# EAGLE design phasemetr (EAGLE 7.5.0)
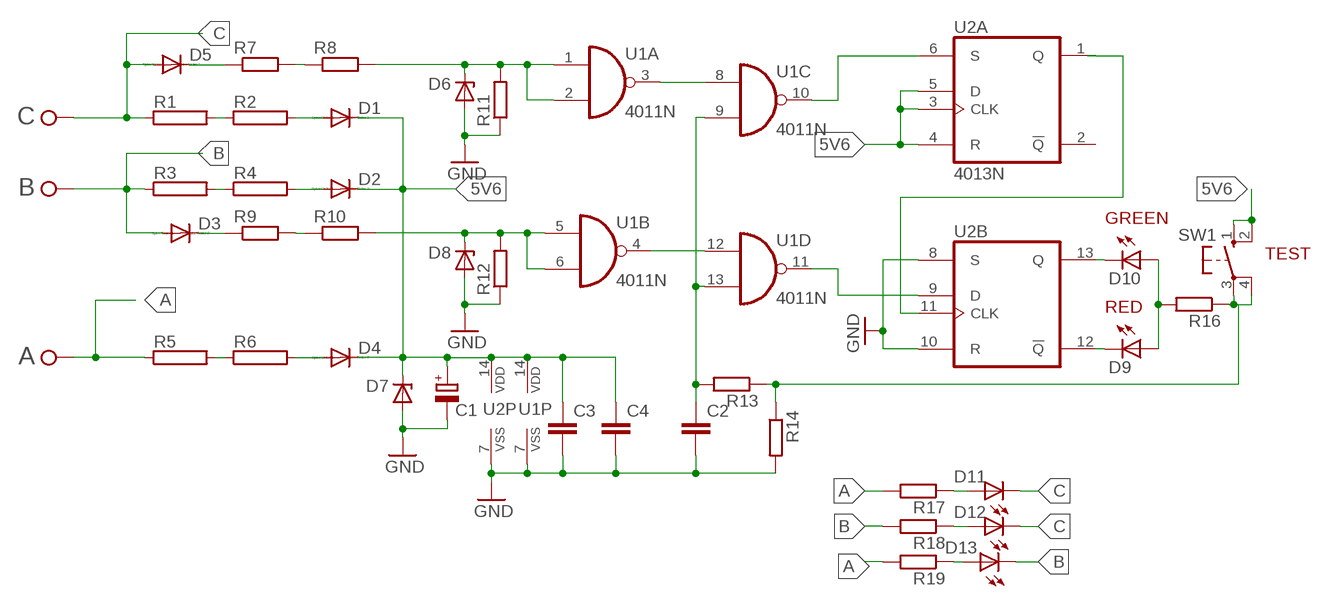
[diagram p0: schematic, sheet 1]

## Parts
A  TPPAD1-20  [P1-20]
B  TPPAD1-20  [P1-20]
C  TPPAD1-20  [P1-20]
C1  CPOL-EUE5-10.5  [E5-10,5]
C2  C-EUC1206  [C1206]
C3  C-EUC1206  [C1206]
C4  C-EUC1206  [C1206]
D1  1N4004  [DO41-10]
D2  1N4004  [DO41-10]
D3  1N4004  [DO41-10]
D4  1N4004  [DO41-10]
D5  1N4004  [DO41-10]
D6  ZY  [P1Z12]
D7  ZY  [P1Z12]
D8  ZY  [P1Z12]
D9  LED5MM  [LED5MM]
D10  LED5MM  [LED5MM]
D11  LED5MM  [LED5MM]
D12  LED5MM  [LED5MM]
D13  LED5MM  [LED5MM]
R1  RRWM8X34  [RWM8X34]
R2  RRWM8X34  [RWM8X34]
R3  RRWM8X34  [RWM8X34]
R4  RRWM8X34  [RWM8X34]
R5  RRWM8X34  [RWM8X34]
R6  RRWM8X34  [RWM8X34]
R7  R-EU_0309/12  [0309/12]
R8  R-EU_0309/12  [0309/12]
R9  R-EU_0309/12  [0309/12]
R10  R-EU_0309/12  [0309/12]
R11  R-EU_0309/12  [0309/12]
R12  R-EU_0309/12  [0309/12]
R13  R-EU_0309/12  [0309/12]
R14  R-EU_0309/12  [0309/12]
R16  R-EU_0309/12  [0309/12]
R17  R-EU_0309/12  [0309/12]
R18  R-EU_0309/12  [0309/12]
R19  R-EU_0309/12  [0309/12]
SW1  10-XX  [B3F-10XX]
U1  4011N  [DIL14]
U2  4013N  [DIL14]

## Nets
5V6: C1.+ C3.1 C4.1 D1.C D2.C D4.C D7.C SW1.1(S) SW1.2(S1) U1.14(P:VDD) U2.3(A:CLK) U2.4(A:R) U2.5(A:D) U2.14(P:VDD)
A: A.TP R5.1 R17.2 R19.2
B: B.TP D3.A D13.K(C) R3.1 R18.2
C: C.TP D5.A D11.K(C) D12.K(C) R1.1
GND: C1.- C2.2 C3.2 C4.2 D6.A D7.A D8.A R11.1 R12.1 R14.2 U1.7(P:VSS) U2.7(P:VSS) U2.8(B:S) U2.10(B:R)
N$2: D5.C R7.1
N$3: D11.A R17.1
N$4: R1.2 R2.1
N$5: D1.A R2.2
N$6: D2.A R4.2
N$7: R3.2 R4.1
N$9: R5.2 R6.1
N$10: D4.A R6.2
N$11: R7.2 R8.1
N$12: D3.C R9.1
N$13: R9.2 R10.1
N$14: D9.A D10.A R16.2
N$15: D6.C R8.2 R11.2 U1.1(A:I0) U1.2(A:I1)
N$16: U1.3(A:O) U1.8(C:I0)
N$17: U1.10(C:O) U2.6(A:S)
N$18: D8.C R10.2 R12.2 U1.5(B:I0) U1.6(B:I1)
N$20: U1.4(B:O) U1.12(D:I0)
N$21: C2.1 R13.2 U1.9(C:I1) U1.13(D:I1)
N$22: U1.11(D:O) U2.9(B:D)
N$23: U2.11(B:CLK)
N$24: D10.K(C) U2.13(B:Q)
N$25: D9.K(C) U2.12(B:!Q)
N$26: R13.1 R14.1 R16.1 SW1.3(P) SW1.4(P1)
N$27: D12.A R18.1
N$29: D13.A R19.1
Unconnected: U2.1(A:Q) U2.2(A:!Q)

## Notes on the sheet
- GREEN
- TEST
- RED

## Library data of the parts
A B C = testpad:TP: Test pad
C1 = rcl:CPOL-EU: POLARIZED CAPACITOR, European symbol
C2-C4 = rcl:C-EU: CAPACITOR, European symbol
D1-D5 = diode:1N4004: DIODE
D6-D8 = diode:ZY: Z DIODE
D9-D13 = led:LED: LED
R1-R6 = resistor-power:R: Power Resitor; OC_FARNELL: unknown; OC_NEWARK: unknown
R7-R14 R16-R19 = rcl:R-EU_: RESISTOR, European symbol
SW1 = switch-omron:10-XX: OMRON SWITCH; MPN: B3F-1000; OC_FARNELL: 176432; OC_NEWARK: 36M3542
U1 = 40xx:4011: Quad 2-input NAND
U2 = 40xx:4013: Dual D FLIP FLOP, set/reset

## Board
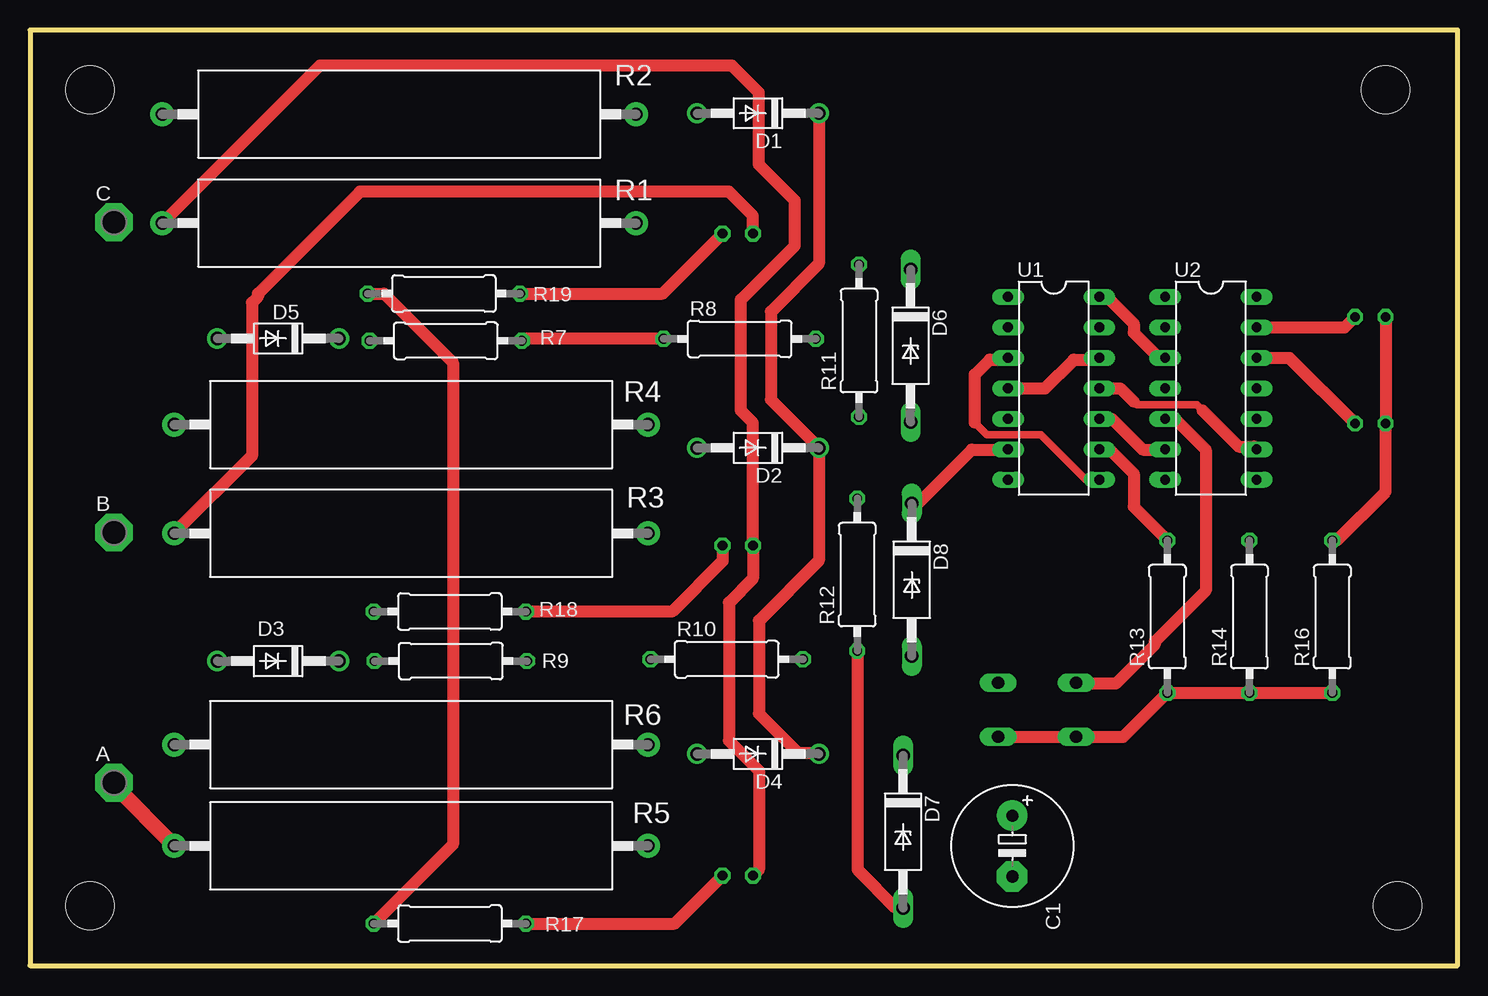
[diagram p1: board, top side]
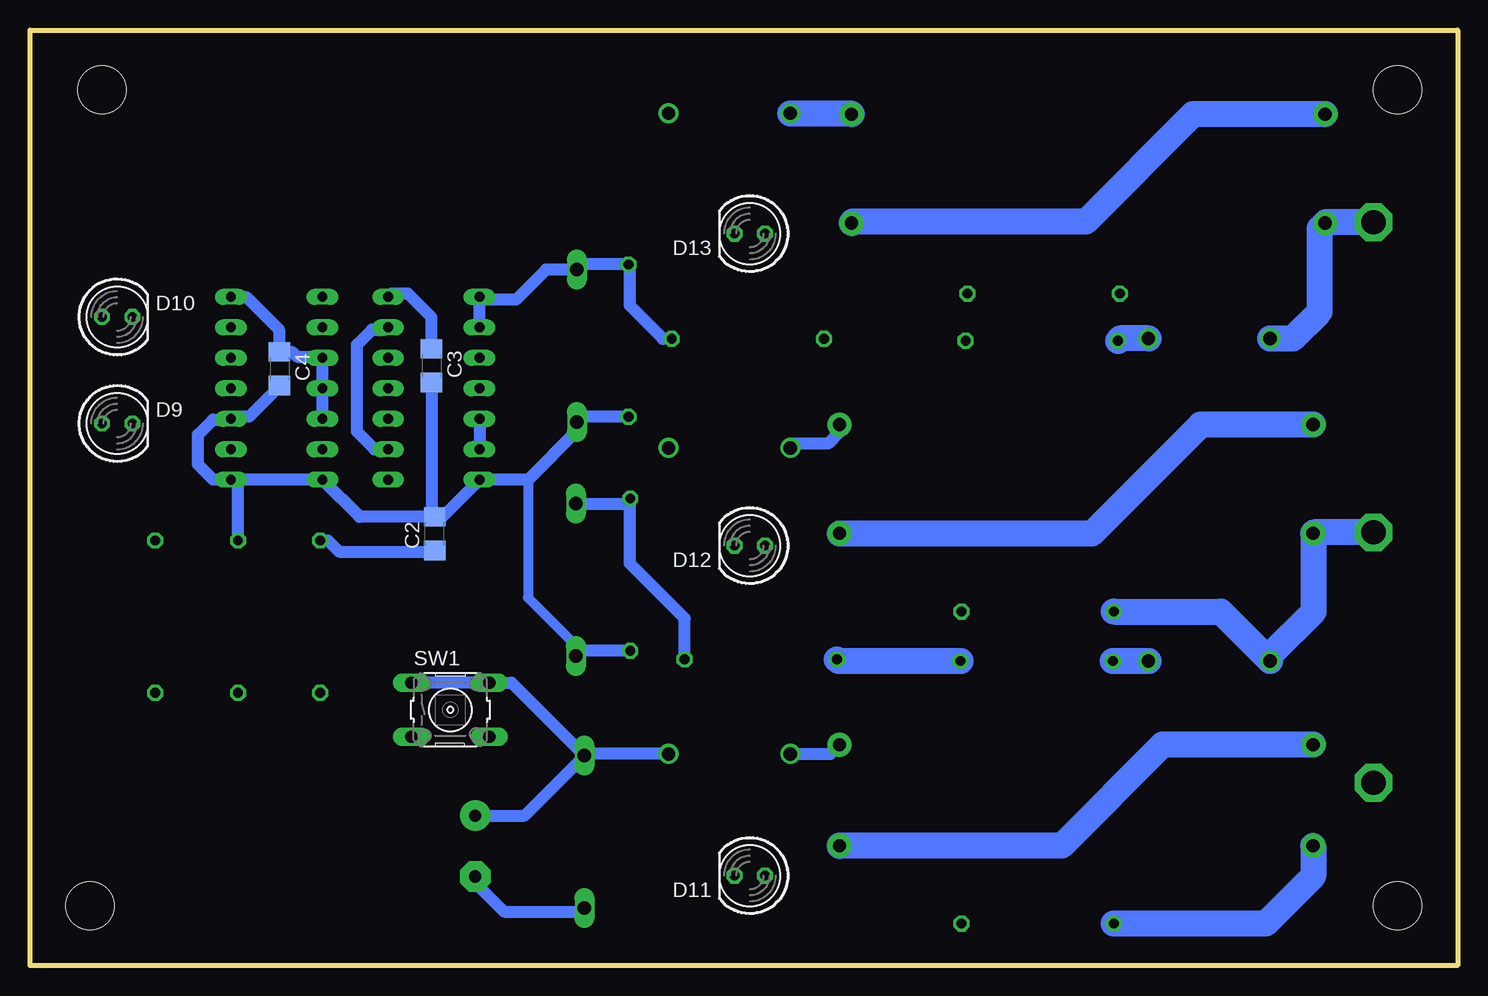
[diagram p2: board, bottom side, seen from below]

Size 119 x 77.97 mm. Coordinates in mm from the lower left corner, seen from the top.
Outline: 0,0 119,0 119,77.97 0,77.97 0,0
Copper layers (1*16): Top 0.035mm / dielectric 1.5mm / Bottom 0.035mm
Design rules "default": minimum track width 10mil, minimum drill 24mil, track to track 8mil, track to pad 8mil, pad to pad 8mil, via to via 8mil, smd to smd 8mil, copper to edge 40mil, drill to drill 8mil, minimum pad ring 10mil, minimum via ring 8mil, stop-mask expansion 4mil, vias tented up to drill 0mil, thermal gap 10mil
Holes 4 mm at 5,73 5,5 114,5 113,73

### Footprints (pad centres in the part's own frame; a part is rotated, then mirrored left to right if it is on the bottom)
P1-20 = drill 2.007 pad 3.15 octagon: TP 0,0
E5-10,5 = drill 1.016 pad 2.54: + -2.54,0 | drill 1.016 pad 2.54 octagon: - 2.54,0
C1206 = smd 1.6 x 1.8: 1 -1.4,0; 2 1.4,0
DO41-10 = drill 1.118: A 5.08,0; C -5.08,0
P1Z12 = drill 1.118 long: A 6.35,0; C -6.35,0
LED5MM = drill 0.813 octagon: A -1.27,0; K 1.27,0
RWM8X34 = drill 1.1 pad 2: 1 -19.74,0; 2 19.74,0
0309/12 = drill 0.813 octagon: 1 -6.35,0; 2 6.35,0
B3F-10XX = drill 1.016 long: 1 -3.251,2.261; 2 3.251,2.261; 3 -3.251,-2.261; 4 3.251,-2.261
DIL14 = drill 0.813 long: 1 -7.62,-3.81; 2 -5.08,-3.81; 3 -2.54,-3.81; 4 0,-3.81; 5 2.54,-3.81; 6 5.08,-3.81; 7 7.62,-3.81; 8 7.62,3.81; 9 5.08,3.81; 10 2.54,3.81; 11 0,3.81; 12 -2.54,3.81; 13 -5.08,3.81; 14 -7.62,3.81

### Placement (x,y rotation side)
A  7,15.25 0 top
B  7,36.1 0 top
C  7,61.95 0 top
C1  81.89,9.96 270 top
C2  85.26,36 90 bottom
C3  85.53,50 270 bottom
C4  98.2,49.75 270 bottom
D1  60.69,71.03 180 top
D2  60.69,43.15 180 top
D3  20.69,25.38 180 top
D4  60.69,17.64 180 top
D5  20.69,52.26 180 top
D6  73.4,51.65 270 top
D7  72.78,11.15 270 top
D8  73.5,32.15 270 top
D9  111.73,45.18 0 bottom
D10  111.73,54.06 0 bottom
D11  59,7.5 180 bottom
D12  59,35 180 bottom
D13  59,61 180 bottom
R1  30.78,61.88 0 top
R2  30.78,70.95 0 top
R3  31.78,36.02 0 top
R4  31.78,45.09 0 top
R5  31.78,9.98 0 top
R6  31.78,18.41 0 top
R7  34.66,52.07 0 top
R8  59.16,52.23 0 top
R9  35.08,25.38 0 top
R10  58.08,25.53 0 top
R11  69.11,52.08 90 top
R12  68.96,32.58 90 top
R13  94.81,29.08 90 top
R14  101.66,29.08 90 top
R16  108.56,29.08 90 top
R17  35,3.5 180 top
R18  35,29.5 180 top
R19  34.5,56 180 top
SW1  83.96,21.32 0 bottom
U1  85.34,48.11 270 top
U2  98.44,48.11 270 top

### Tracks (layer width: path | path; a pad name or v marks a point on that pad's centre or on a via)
5V6
  Top 1.016: U1.14 89.77,55.73 92,53.5 92,52.75 94,50.75 94.53,50.75 U2.3 | U2.5 95.43,45.57 98,43 98,31.25 93.75,27 93.75,26.75 90.5,23.5 87.29,23.5 SW1.1 | D1.C 65.77,58.52 61.75,54.5 61.75,47.17 D2.C 65.77,33.77 60.75,28.75 60.75,21 64,17.75 65.66,17.75 D4.C
  Bottom 1.016: D4.C 72.64,17.64 D7.C | C1.+ 77.78,12.5 D7.C | C3.1 85.53,54.03 87.5,56 88.88,56 U1.14 | U2.5 U2.4 U2.3 94.73,50.75 96.75,50.75 97.15,51.15 C4.1 98.25,51.2 98.25,53 100.98,55.73 U2.14 | D7.C 78.86,23.58 SW1.2 SW1.1
A
  Top 1.016: R19.2 29.5,56 35.25,50.25 35.25,10.1 R17.2
  Top 1.27: A.TP 7,15.02 R5.1
  Bottom 2.184: R5.1 12.04,7.46 16,3.5 R17.2
B
  Top 1.016: D13.K 60.27,62.48 58.25,64.5 27.5,64.5 19,56 19,55.75 18.5,55.25 18.5,42.48 R3.1
  Bottom 2.184: B.TP 11.96,36.1 R3.1 12,35.98 12,29.5 15.61,25.89 D3.A 19.73,29.5 R18.2
C
  Top 1.016: D11.K 60.75,7.98 60.75,16.25 58.25,18.75 58.25,30.25 60.27,32.27 D12.K 60.27,45.23 59.25,46.25 59.25,55.5 63.75,60 63.75,63.75 60.75,66.75 60.75,72.75 58.5,75 24.16,75 R1.1
  Bottom 2.184: C.TP 10.97,61.95 R1.1 11.5,61.42 11.5,54.5 13.74,52.26 D5.A
GND
  Top 1.016: D7.A 72.2,4.8 69,8 69,26.19 R12.1
  Bottom 0.813: 77.5,40.5 77.5,30.66 73.07,26.23
  Bottom 1.016: R12.1 73.07,26.23 D8.A | C1.- 81.89,6.89 79.5,4.5 73.08,4.5 D7.A | R11.1 72.97,45.73 D6.A 73.4,44.6 77.5,40.5 U1.7 84.62,37.4 C2.2 | C2.2 91.54,37.4 U2.7 101.75,40.49 | 101.75,40.49 U2.8 103.74,40.49 105,41.75 105,44.25 103.75,45.5 102.32,45.5 U2.10 102.07,45.75 100.75,45.75 98.2,48.3 C4.2 | C3.2 85.53,37.67 C2.2 | R14.2 101.66,40.4 101.75,40.49
N$2
  Bottom 2.184: D5.C 28.12,52.26 R7.1
N$3
  Top 1.016: R17.1 53.73,3.5 D11.A
N$4
  Bottom 2.184: R2.1 22.05,70.95 31,62 50.4,62 R1.2
N$5
  Bottom 2.184: D1.A 50.6,71.03 R2.2
N$6
  Bottom 1.016: R4.2 51.52,44.48 52.5,43.5 55.26,43.5 D2.A
N$7
  Bottom 2.184: R4.1 21.41,45.09 30.5,36 51.5,36 R3.2
N$9
  Bottom 2.184: R6.1 24.59,18.41 33,10 51.5,10 R5.2
N$10
  Bottom 1.016: D4.A 52.29,17.64 R6.2
N$11
  Top 1.016: R8.1 41.17,52.23 R7.2
N$12
  Bottom 2.184: D3.C R9.1
N$13
  Bottom 2.184: R9.2 51.58,25.38 R10.1
N$14
  Top 1.016: D10.A D9.A 113,39.5 108.93,35.43 R16.2
N$15
  Bottom 1.016: R8.2 66.23,52.23 69,55 69,58.32 R11.2 73.57,58.43 74,58 D6.C 76,58 78.5,55.5 81.3,55.5 U1.1 U1.2
N$16
  Top 0.61: U1.8 88.01,40.49 84.25,44.25 79.75,44.25 78.75,45.25
  Top 1.016: 78.75,45.25 78.75,49.25 80,50.5 81.38,50.5 U1.3
N$17
  Top 1.016: U1.10 90.18,45.57 92.75,43 94.6,43 U2.6
N$18
  Top 1.016: D8.C 74,38.5 78.5,43 81.5,43 U1.6
  Bottom 1.016: R10.2 64.43,28.93 69,33.5 69,38.89 R12.2 69.39,38.5 D8.C | U1.5 U1.6
N$20
  Top 1.016: U1.4 84.61,48.11 87,50.5 89,50.5 U1.12
N$21
  Top 1.016: U1.9 89.97,43.03 92,41 92,38.24 R13.2
  Bottom 1.016: R13.2 94.18,35.43 93.25,34.5 85.36,34.5 C2.1 | U1.9 90.28,43.03 91.75,44.5 91.75,51.75 90.5,53 89.34,53 U1.13
N$22
  Top 0.61: 92,47 92.25,46.75 97.25,46.75 97.75,46.25
  Top 1.016: U1.11 90.89,48.11 92,47 | 97.75,46.25 100.75,43.25 102.03,43.25 U2.9
N$24
  Top 1.016: U2.13 109.59,53.19 D10.K
N$25
  Top 1.016: U2.12 104.99,50.65 D9.K
N$26
  Top 1.016: 94.64,22.56 R13.1 | R13.1 R14.1 R16.1 | R13.1 91.14,19.06 SW1.3 SW1.4
N$27
  Top 1.016: D12.A 57.73,33.73 53.5,29.5 R18.1
N$29
  Top 1.016: R19.1 52.73,56 D13.A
